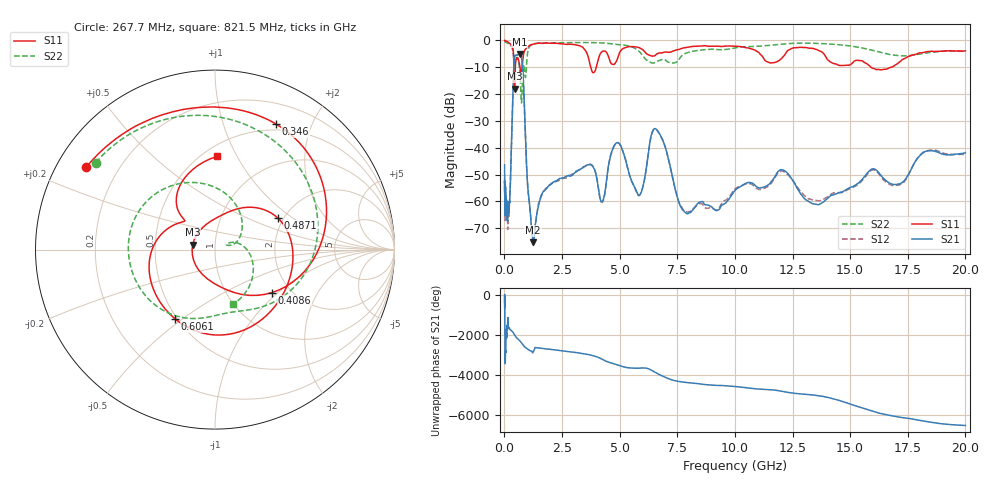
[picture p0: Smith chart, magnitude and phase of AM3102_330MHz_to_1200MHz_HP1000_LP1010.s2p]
! Date/Time: Tue, Sep 11, 2018 5:17 PM
! Network Analyzer: Agilent Technologies E8362B Rev: A.07.50.63
! Sweep from 0.010 to 20.000 GHz, 1601 Points, Sweep Type: LOG
! Power Supply: 4.949 V, 0.001 A
# Hz S DB R 50
!freq MagS11 AngS11 MagS21 AngS21 MagS12 AngS12 MagS22 AngS22
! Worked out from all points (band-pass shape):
!   1601 points, 10 MHz to 20 GHz, reference 50 ohm
!   highest |S21| = -4.98 dB at 663.4 MHz (marker M1); lowest = -75.2 dB at 1.242 GHz (marker M2)
!   |S21| within 3 dB of the highest: 420.5 MHz to 771 MHz (350.5 MHz wide, 58.8 % of centre)
!   lowest |S11| = -17.9 dB at 440.9 MHz (marker M3), VSWR 1.29, Z = 38.9 + j2.16 ohm
!   |S11| at or under -10 dB: 676 MHz to 769.5 MHz (93.58 MHz wide, 12.9 % of centre); 3.747 GHz to 3.986 GHz (238.8 MHz wide, 6.17 % of centre); 15.91 GHz to 16.77 GHz (860.1 MHz wide, 5.26 % of centre)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
!   |S22| runs from -23.3 to -0.2 dB; largest |S21 - S12| = 0.01
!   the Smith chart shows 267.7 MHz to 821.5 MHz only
!   S11 on the Smith chart (normalised r, x): 267.7 MHz: 0.09, +0.29; 346 MHz: 0.43, +1.51; 408.6 MHz: 1.61, -0.92; 487.1 MHz: 1.87, +0.78; 606.1 MHz: 0.49, -0.47; 821.5 MHz: 0.58, +0.83
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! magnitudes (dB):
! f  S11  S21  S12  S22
! 10 MHz  0.0  -46.4  -52.3  -0.2
! 35.55 MHz  0.0  -62.4  -66.2  -0.4
! 126.4 MHz  -0.4  -65.1  -66.5  -0.9
! 267.7 MHz  -1.4  -51.1  -50.7  -1.7
! 346 MHz  -2.2  -27.2  -27.3  -3.1
! 408.6 MHz  -8.0  -10.0  -10.0  -6.6
! 440.9 MHz  -17.9  -6.1  -6.2  -8.9
! 447.2 MHz  -17.4  -5.8  -5.9  -8.9
! 487.1 MHz  -8.1  -5.5  -5.5  -7.2
! 606.1 MHz  -7.0  -5.2  -5.3  -7.4
! 663.4 MHz  -9.2  -5.0  -5.0  -11.0
! 740 MHz  -12.4  -6.0  -6.1  -23.3
! 821.5 MHz  -5.7  -14.7  -14.8  -9.9
! 1.242 GHz  -1.4  -75.2  -76.7  -1.3
! 1.59 GHz  -1.0  -57.9  -58.4  -0.9
! 3.668 GHz  -7.2  -46.3  -46.1  -0.8
! 4.251 GHz  -4.1  -60.0  -60.3  -0.9
! 4.902 GHz  -6.9  -38.1  -38.2  -1.5
! 5.652 GHz  -2.3  -54.7  -55.0  -2.9
! 6.58 GHz  -5.3  -33.0  -33.1  -8.0
! 7.92 GHz  -2.5  -64.6  -64.0  -4.6
! 20 GHz  -3.9  -41.9  -42.5  -3.9
